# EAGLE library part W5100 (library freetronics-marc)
WIZnet W5100
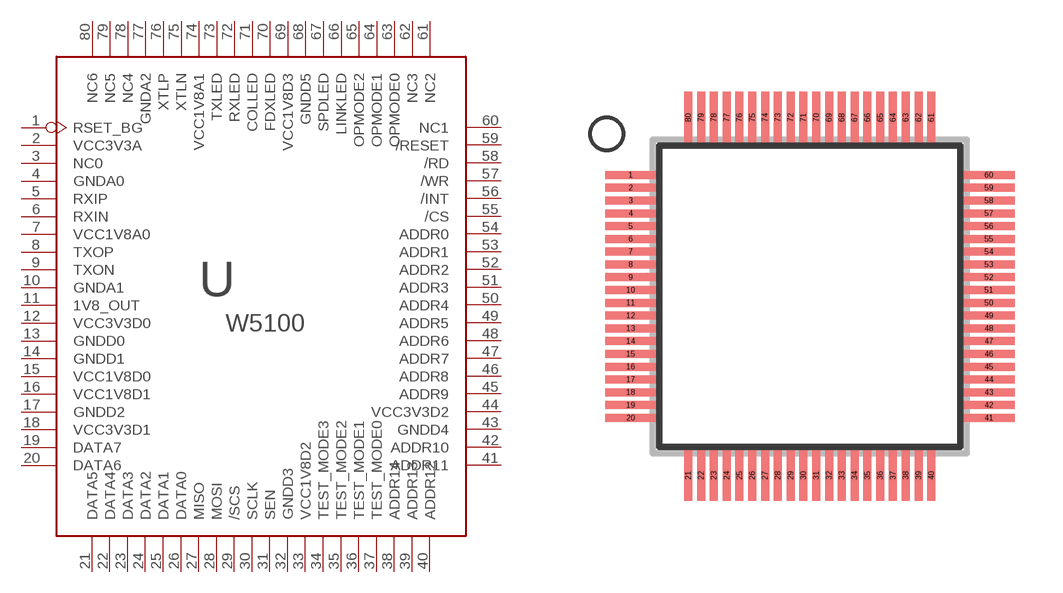
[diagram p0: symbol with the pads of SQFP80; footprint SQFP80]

Designator prefix -

## W5100SQFP80  [SQFP80]
1  RSET_BG
2  VCC3V3A
3  NC0
4  GNDA0
5  RXIP
6  RXIN
7  VCC1V8A0
8  TXOP
9  TXON
10  GNDA1
11  1V8_OUT
12  VCC3V3D0
13  GNDD0
14  GNDD1
15  VCC1V8D0
16  VCC1V8D1
17  GNDD2
18  VCC3V3D1
19  DATA7
20  DATA6
21  DATA5
22  DATA4
23  DATA3
24  DATA2
25  DATA1
26  DATA0
27  MISO
28  MOSI
29  /SCS
30  SCLK
31  SEN
32  GNDD3
33  VCC1V8D2
34  TEST_MODE3
35  TEST_MODE2
36  TEST_MODE1
37  TEST_MODE0
38  ADDR14
39  ADDR13
40  ADDR12
41  ADDR11
42  ADDR10
43  GNDD4
44  VCC3V3D2
45  ADDR9
46  ADDR8
47  ADDR7
48  ADDR6
49  ADDR5
50  ADDR4
51  ADDR3
52  ADDR2
53  ADDR1
54  ADDR0
55  /CS
56  /INT
57  /WR
58  /RD
59  /RESET
60  NC1
61  NC2
62  NC3
63  OPMODE0
64  OPMODE1
65  OPMODE2
66  LINKLED
67  SPDLED
68  GNDD5
69  VCC1V8D3
70  FDXLED
71  COLLED
72  RXLED
73  TXLED
74  VCC1V8A1
75  XTLN
76  XTLP
77  GNDA2
78  NC4
79  NC5
80  NC6

## Footprint SQFP80 (pad centres in mm)
smd 1.6 x 0.25: 1 -5.6,3.8; 2 -5.6,3.4; 3 -5.6,3; 4 -5.6,2.6; 5 -5.6,2.2; 6 -5.6,1.8; 7 -5.6,1.4; 8 -5.6,1; 9 -5.6,0.6; 10 -5.6,0.2; 11 -5.6,-0.2; 12 -5.6,-0.6; 13 -5.6,-1; 14 -5.6,-1.4; 15 -5.6,-1.8; 16 -5.6,-2.2; 17 -5.6,-2.6; 18 -5.6,-3; 19 -5.6,-3.4; 20 -5.6,-3.8; 41 5.6,-3.8; 42 5.6,-3.4; 43 5.6,-3; 44 5.6,-2.6; 45 5.6,-2.2; 46 5.6,-1.8; 47 5.6,-1.4; 48 5.6,-1; 49 5.6,-0.6; 50 5.6,-0.2; 51 5.6,0.2; 52 5.6,0.6; 53 5.6,1; 54 5.6,1.4; 55 5.6,1.8; 56 5.6,2.2; 57 5.6,2.6; 58 5.6,3; 59 5.6,3.4; 60 5.6,3.8
smd 0.25 x 1.6: 21 -3.8,-5.6; 22 -3.4,-5.6; 23 -3,-5.6; 24 -2.6,-5.6; 25 -2.2,-5.6; 26 -1.8,-5.6; 27 -1.4,-5.6; 28 -1,-5.6; 29 -0.6,-5.6; 30 -0.2,-5.6; 31 0.2,-5.6; 32 0.6,-5.6; 33 1,-5.6; 34 1.4,-5.6; 35 1.8,-5.6; 36 2.2,-5.6; 37 2.6,-5.6; 38 3,-5.6; 39 3.4,-5.6; 40 3.8,-5.6; 61 3.8,5.6; 62 3.4,5.6; 63 3,5.6; 64 2.6,5.6; 65 2.2,5.6; 66 1.8,5.6; 67 1.4,5.6; 68 1,5.6; 69 0.6,5.6; 70 0.2,5.6; 71 -0.2,5.6; 72 -0.6,5.6; 73 -1,5.6; 74 -1.4,5.6; 75 -1.8,5.6; 76 -2.2,5.6; 77 -2.6,5.6; 78 -3,5.6; 79 -3.4,5.6; 80 -3.8,5.6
